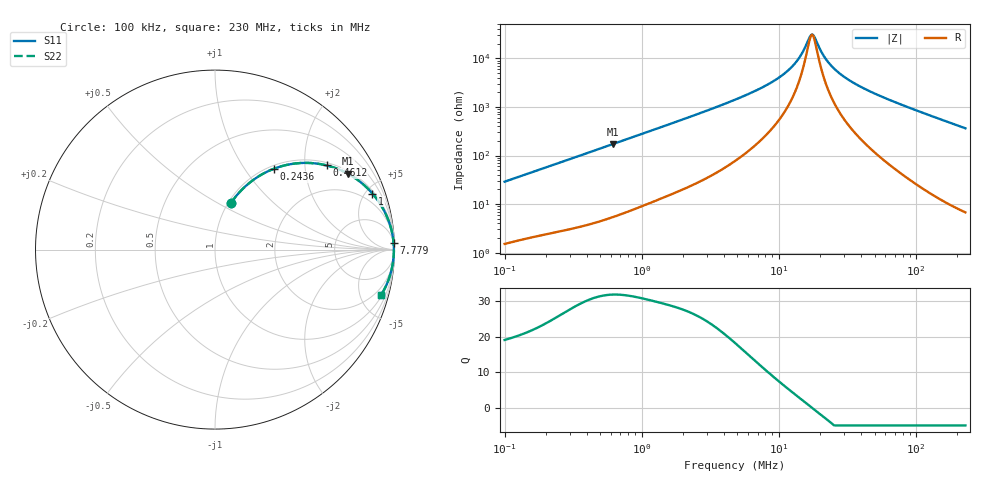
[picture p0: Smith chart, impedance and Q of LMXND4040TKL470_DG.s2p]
! LMXND4040TKL470_DG  S-PARAMETER MODEL  ( General Type )
! Model Generated by TAIYO YUDEN Corporation (http://www.ty-top.com)
! Version 1.0
! TAIYO YUDEN Control No. 191023NI43SB-FBB
! Copyright(c) 2019 TAIYO YUDEN CO.,LTD. All Rights Reserved.
! Product Description (link to TY-COMPAS)
! https://ds.yuden.co.jp/TYCOMPAS/or/detail?pn=LMXND4040TKL470MDG&u=M
! Products Name : Inductors
! Characteristics :
!  Inductance : 47 uH , SRF(min) : 10 MHz , DC Resistance(max) : 0.78 Ohm
!  Rated Current : Saturation :600 mA , Temp Rise : 440 mA
!  Case Size : 4.0 x 4.0 / 0.157 x 0.157 [mm/inch] , Thickness : 1.8 / 0.071 [mm/inch]
!  (Conditions: Temperature = 25 degC , DC Bias Current/Voltage = 0A / 0V)
! External Node Assignments :
!  1  o---GGG---o  2
! GND o---------o GND
! Frequency Range : 0.1MHz  -  229.966873MHz  [ 402 STEP ]
# MHz S RI R 50
! Freq[MHz].  S11 Real  S11 Imag  S21 Real  S21 Imag  S12 Real  S12 Imag  S22 Real  S22 Imag
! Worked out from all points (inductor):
!   401 points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, 100 kHz to 230 MHz, reference 50 ohm
!   read as one part in series: L = 45.6 uH near 103.9 kHz
!   highest Q = 31.9 at 616.6 kHz (marker M1), where L = 44.4 uH
!   self-resonance near 17.2 MHz
!   S11 on the Smith chart (normalised r, x): 100 kHz: 1.03, +0.58; 243.6 kHz: 1.05, +1.38; 461.2 kHz: 1.08, +2.58; 1 MHz: 1.18, +5.55; 7.779 MHz: 6, +52; 230 MHz: 1.14, -7.27
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0.1  0.0887 0.2593  0.9113 -0.2593  0.9113 -0.2593  0.0887 0.2593
0.159111  0.1819 0.3636  0.8181 -0.3636  0.8181 -0.3636  0.1819 0.3636
0.243552  0.3277 0.4503  0.6723 -0.4503  0.6723 -0.4503  0.3277 0.4503
0.365661  0.5127 0.4832  0.4873 -0.4832  0.4873 -0.4832  0.5127 0.4832
0.461242  0.6213 0.4692  0.3787 -0.4692  0.3787 -0.4692  0.6213 0.4692
0.616583  0.7409 0.4227  0.2591 -0.4227  0.2591 -0.4227  0.7409 0.4227
1.00022  0.8774 0.3121  0.1226 -0.3121  0.1226 -0.3121  0.8774 0.3121
1.337081  0.9249 0.2473  0.0751 -0.2473  0.0751 -0.2473  0.9249 0.2473
4.889189  0.9914 0.0685  0.00858 -0.0685  0.00858 -0.0685  0.9914 0.0685
7.779232  0.9951 0.0377  0.00486 -0.0377  0.00486 -0.0377  0.9951 0.0377
10.19988  0.9961 0.0237  0.00388 -0.0237  0.00388 -0.0237  0.9961 0.0237
12.61946  0.9965 0.0139  0.00345 -0.0139  0.00345 -0.0139  0.9965 0.0139
14.17313  0.9967 0.0089  0.00331 -0.0089  0.00331 -0.0089  0.9967 0.0089
16.86954  0.9968 0.00155  0.00321 -0.00155  0.00321 -0.00155  0.9968 0.00155
17.53523  0.9968 -6.95e-05  0.00321 6.95e-05  0.00321 6.95e-05  0.9968 -6.95e-05
18.2272  0.9968 -0.00169  0.00321 0.00169  0.00321 0.00169  0.9968 -0.00169
20.47127  0.9968 -0.00657  0.00324 0.00657  0.00324 0.00657  0.9968 -0.00657
22.1188  0.9967 -0.00987  0.00329 0.00987  0.00329 0.00987  0.9967 -0.00987
27.36575  0.9964 -0.0193  0.00356 0.0193  0.00356 0.0193  0.9964 -0.0193
38.76879  0.9954 -0.0368  0.00457 0.0368  0.00457 0.0368  0.9954 -0.0368
64.11956  0.9917 -0.0705  0.00831 0.0705  0.00831 0.0705  0.9917 -0.0705
229.9669  0.9257 -0.2532  0.0743 0.2532  0.0743 0.2532  0.9257 -0.2532
